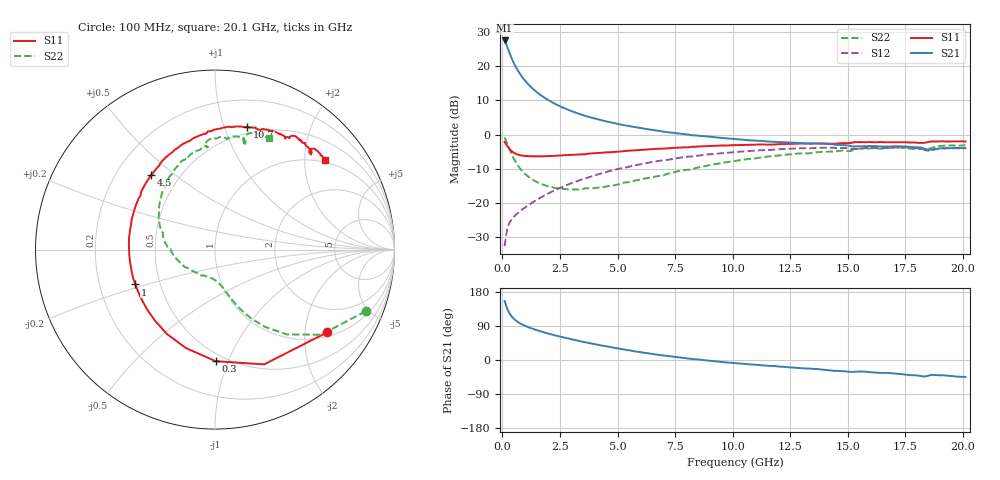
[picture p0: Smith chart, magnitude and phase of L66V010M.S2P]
!  Infineon Technologies AG
! BFR380L3 , PF131585-7, No.6, Th 09.10.01, soldered on pcb-board, measured with PP GSG850
!  Vce=6.0 V,  Ic=10.0 mA
! Common Emitter S-Parameters:  15. November 2001
#  GHz  S  MA  R  50
! f  S11  S21  S12  S22
! GHz  Mag  Ang  Mag  Ang  Mag  Ang  Mag  Ang
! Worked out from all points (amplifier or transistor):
!   201 points, 100 MHz to 20.1 GHz, reference 50 ohm
!   highest |S21| = 27.6 dB at 100 MHz (marker M1)
!   |S21| within 3 dB of that: start of sweep to 275.1 MHz
!   unconditionally stable (mu >= 1): 1.915 GHz to 4.429 GHz
!   at 3.4 GHz: K = 1.03, MAG = 8.6 dB, |S12| = -13.3 dB
!   at 10.1 GHz: K = 0.93, MSG = 1.9 dB, |S12| = -5.1 dB
!   at 20.1 GHz: K = 0.99, MSG = 0.0 dB, |S12| = -4.0 dB
!   S11 on the Smith chart (normalised r, x): 100 MHz: 1.12, -2.60; 300 MHz: 0.44, -0.90; 1 GHz: 0.36, -0.18; 4.5 GHz: 0.35, +0.41; 10.7 GHz: 0.44, +1.20; 20.1 GHz: 0.95, +2.51
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0.1  0.7756 -36.5  24.04 155.7  0.02297 71.7  0.9073 -22.3
0.2  0.6956 -66.8  19.88 137.2  0.03965 59.7  0.7574 -38.8
0.3  0.6217 -89.7  16.16 124.5  0.05007 53.7  0.6208 -49.6
0.4  0.572 -106.5  13.33 115.5  0.05675 50.5  0.5167 -56.8
0.5  0.5412 -119.6  11.23 108.7  0.06203 49.3  0.4407 -61.8
0.6  0.5188 -129.9  9.645 103.6  0.06685 49.4  0.3846 -65.4
0.7  0.5045 -138.4  8.443 99.4  0.07139 49.6  0.3417 -68.1
0.8  0.4949 -145.2  7.487 95.7  0.0761 50.4  0.3086 -70.3
1  0.484 -156.3  6.108 89.8  0.08537 52.0  0.262 -73.8
1.2  0.4801 -165.0  5.153 84.9  0.09498 53.5  0.2306 -76.8
1.4  0.478 -172.0  4.462 80.7  0.1051 54.7  0.2089 -79.6
1.6  0.4781 -178.0  3.934 76.7  0.1155 55.8  0.1935 -82.4
1.9  0.4813 174.4  3.353 71.4  0.1316 56.6  0.1776 -86.7
2.6  0.4943 159.8  2.51 60.4  0.1702 56.8  0.1599 -98.6
3.5  0.5121 144.5  1.924 47.9  0.2226 54.5  0.1583 -114.8
4.5  0.5469 130.7  1.563 36.0  0.281 50.4  0.1722 -136.5
6.8  0.6182 105.1  1.129 13.4  0.4111 37.0  0.2461 -179.2
10.1  0.6984 79.1  0.8563 -8.4  0.5534 15.3  0.4105 138.2
10.7  0.7048 75.2  0.8241 -11.3  0.5731 11.2  0.4383 131.1
13.5  0.7374 60.8  0.7395 -23.5  0.6327 -6.6  0.5412 105.4
16.8  0.7698 48.3  0.6694 -34.3  0.6403 -23.5  0.636 81.6
20.1  0.79 38.9  0.6311 -44.9  0.631 -37.6  0.694 64.1
